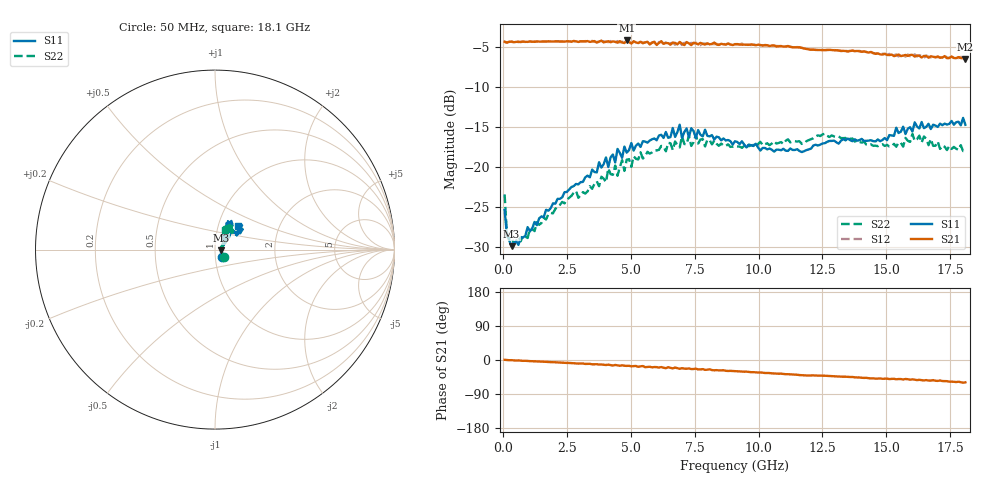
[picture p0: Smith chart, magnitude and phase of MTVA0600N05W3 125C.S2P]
! Network Analyzer HP8720D.06.14 Serial No. US36140669
!  8 Jul 2005  13:40:53
! Frequency  S11  S21  S12  S22
# HZ  S  DB R 50
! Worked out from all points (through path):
!   201 points, 50 MHz to 18.1 GHz, reference 50 ohm
!   highest |S21| = -4.16 dB at 4.833 GHz (marker M1); lowest = -6.5 dB at 18.1 GHz (marker M2)
!   group delay of S21, straight-line fit = 9.22 ps
!   lowest |S11| = -29.9 dB at 320.8 MHz (marker M3), VSWR 1.07, Z = 53.3 - j0.335 ohm
!   |S11| at or under -10 dB: start of sweep to end of sweep
!   |S22| runs from -29.6 to -15.8 dB; largest |S21 - S12| = 0.028
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5e7  -25.40 -46.0  -4.31 0.6  -4.35 0.7  -23.44 -39.4
1.4025e8  -28.52 -26.8  -4.43 -0.1  -4.42 -0.1  -28.26 -24.7
3.2075e8  -29.92 -5.6  -4.30 -0.4  -4.34 -0.3  -28.85 -6.5
9.525e8  -27.53 17.9  -4.34 -2.5  -4.28 -2.7  -28.89 18.4
3.1185e9  -21.87 41.2  -4.28 -9.1  -4.32 -9.5  -23.16 48.0
4.021e9  -18.81 47.5  -4.34 -13.2  -4.31 -12.4  -21.91 51.4
4.11125e9  -20.01 47.9  -4.26 -12.2  -4.37 -13.3  -20.19 52.3
4.29175e9  -18.44 53.7  -4.27 -14.6  -4.41 -13.6  -20.98 49.0
4.382e9  -19.44 48.4  -4.33 -13.1  -4.38 -14.4  -19.83 55.1
4.47225e9  -17.74 45.8  -4.44 -14.2  -4.24 -13.7  -21.11 58.7
4.83325e9  -18.21 55.8  -4.16 -15.5  -4.37 -15.9  -19.10 50.4
6.09675e9  -16.07 55.0  -4.46 -19.9  -4.36 -19.9  -17.86 56.5
6.7285e9  -16.23 62.0  -4.47 -19.9  -4.71 -20.5  -16.81 54.0
6.909e9  -14.71 60.3  -4.35 -23.3  -4.41 -21.8  -17.56 54.2
6.99925e9  -16.37 60.2  -4.56 -21.6  -4.73 -23.3  -16.15 55.8
7.36025e9  -15.15 56.7  -4.75 -23.9  -4.46 -23.3  -17.37 60.0
7.54075e9  -16.38 58.9  -4.52 -22.8  -4.44 -25.4  -15.97 58.9
9.075e9  -16.78 62.6  -4.63 -29.4  -4.61 -29.6  -17.38 50.4
1.21435e10  -17.32 49.2  -5.31 -40.6  -5.26 -40.9  -16.40 55.8
1.512175e10  -16.01 36.0  -5.99 -50.4  -5.84 -50.1  -17.45 61.8
1.602425e10  -15.57 36.7  -5.97 -51.1  -6.14 -53.2  -15.87 59.2
1.81e10  -14.72 44.5  -6.49 -58.9  -6.65 -59.8  -18.04 62.6
